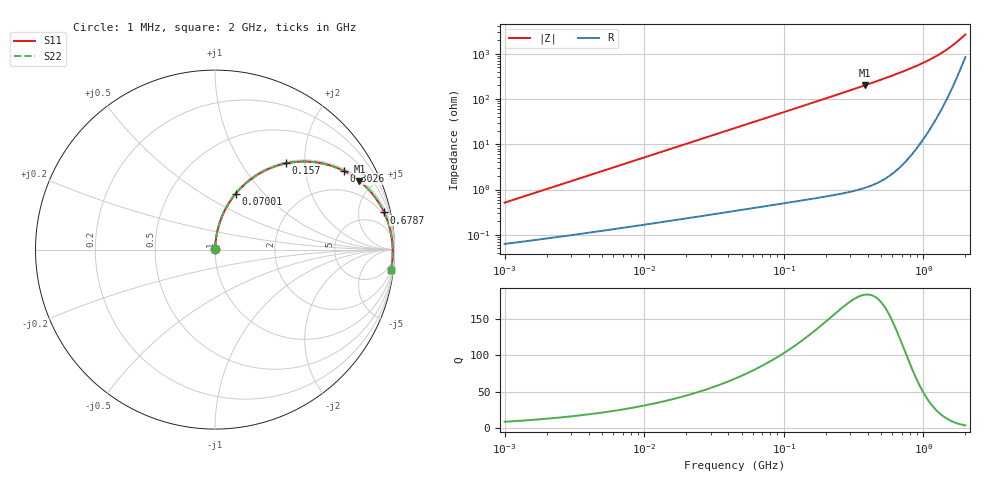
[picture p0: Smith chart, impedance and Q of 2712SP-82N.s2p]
# MHz  S  MA  R  50
!Freq  MagS11  AngS11  MagS21  AngS21  MagS12  AngS12  MagS22  AngS22
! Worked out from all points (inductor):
!   801 points, 1 MHz to 2 GHz, reference 50 ohm
!   read as one part in series: L = 81.1 nH near 1.039 MHz
!   highest Q = 184 at 380.1 MHz (marker M1), where L = 83.5 nH
!   S11 on the Smith chart (normalised r, x): 1 MHz: 1.00, +0.01; 70.01 MHz: 1.01, +0.71; 157 MHz: 1.03, +1.61; 302.6 MHz: 1.08, +3.21; 678.7 MHz: 1.49, +8.98; 2 GHz: 2, -17
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1  0.005099 82.6  0.9994 -0.3  0.9994 -0.3  0.005099 82.6
3.573795  0.01811 85.6  0.9988 -1.0  0.9988 -1.0  0.0181 85.6
7.152559  0.03617 85.6  0.9979 -2.1  0.9979 -2.1  0.03617 85.6
12.65119  0.06384 84.6  0.9961 -3.7  0.9961 -3.7  0.06384 84.6
24.8432  0.1245 81.6  0.9897 -7.2  0.9897 -7.2  0.1245 81.6
44.78507  0.2206 76.3  0.9721 -12.9  0.9721 -12.9  0.2206 76.3
70.00699  0.3332 69.6  0.939 -19.7  0.939 -19.7  0.3332 69.6
85.4724  0.3962 65.8  0.914 -23.6  0.914 -23.6  0.3962 65.8
104.3543  0.4662 61.3  0.8802 -28.1  0.8802 -28.1  0.4662 61.3
127.4075  0.5413 56.3  0.8362 -33.2  0.8362 -33.2  0.5412 56.3
157.0389  0.622 50.6  0.7782 -39.0  0.7782 -39.0  0.6219 50.6
160.0527  0.6293 50.0  0.7724 -39.5  0.7724 -39.5  0.6292 50.0
219.0188  0.7436 40.8  0.6639 -48.8  0.6639 -48.8  0.7434 40.8
302.5713  0.8399 31.5  0.538 -58.2  0.538 -58.2  0.8398 31.5
380.0981  0.891 25.4  0.4494 -64.3  0.4494 -64.3  0.8908 25.4
464.0665  0.9245 20.5  0.3763 -69.2  0.3763 -69.2  0.9243 20.5
566.5845  0.949 16.0  0.3094 -73.6  0.3094 -73.6  0.9488 16.0
678.7245  0.965 12.4  0.2549 -77.2  0.2549 -77.2  0.9647 12.4
955.6426  0.9831 6.1  0.1669 -82.8  0.1669 -82.8  0.9828 6.1
1258.933  0.9893 1.5  0.1088 -86.0  0.1088 -86.0  0.9891 1.5
1551.726  0.9902 -2.0  0.07173 -86.3  0.07173 -86.3  0.9901 -2.0
2000  0.9873 -6.8  0.03704 -78.3  0.03704 -78.3  0.9875 -6.8
